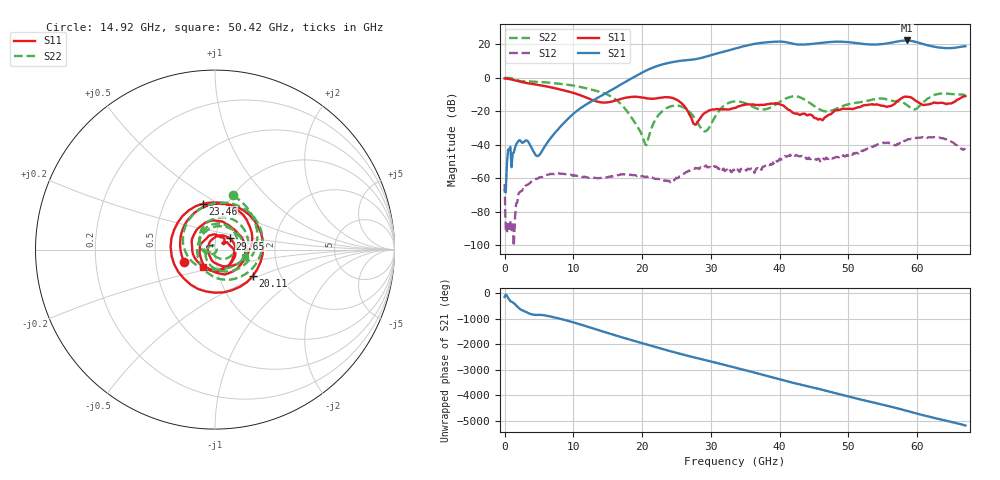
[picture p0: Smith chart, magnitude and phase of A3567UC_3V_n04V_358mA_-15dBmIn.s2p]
! MARKI MICROWAVE INC.
! Date:  4/20/2021
! Model Number:  A-3567UC
! Description:  2-port Small Signal S-parameter data for A-3567UC
! Frequency Range:  10 MHz to 67 GHz
! Port Configuration:  PORT 1: Input
!  PORT 2: Output
! Bias Condition: Vd = +3V, Vg = -0.4V, Id = 358mA
! A-3567UC s2p files are only valid for small signal conditions (below -10 dBm input power)
# Hz S  dB  R 50
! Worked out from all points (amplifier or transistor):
!   401 points, 10 MHz to 67 GHz, reference 50 ohm
!   highest |S21| = 22.3 dB at 58.46 GHz (marker M1)
!   |S21| within 3 dB of that: 35.21 GHz to 61.62 GHz (26.41 GHz wide, 54.5 % of centre)
!   unconditionally stable (mu >= 1): 178.7 MHz to end of sweep
!   at 11.06 GHz: K = 2250.85, MAG = -16.2 dB, |S12| = -58.7 dB
!   at 33.51 GHz: K = 40.23, MAG = 17.7 dB, |S12| = -56.0 dB
!   at 67 GHz: K = 6.21, MAG = 19.6 dB, |S12| = -42.2 dB
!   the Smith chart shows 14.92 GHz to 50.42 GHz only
!   S11 on the Smith chart (normalised r, x): 14.92 GHz: 0.70, -0.10; 20.11 GHz: 1.44, -0.46; 23.46 GHz: 0.77, +0.42; 29.65 GHz: 1.17, +0.15; 50.42 GHz: 0.86, -0.17
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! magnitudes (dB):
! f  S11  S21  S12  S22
! 10 MHz  -0.4  -67.1  -63.4  0.0
! 512.4 MHz  -0.6  -42.9  -85.6  0.0
! 2.02 GHz  -2.0  -37.7  -69.4  -1.6
! 4.867 GHz  -4.2  -46.7  -60.0  -2.4
! 11.23 GHz  -10.7  -17.6  -59.0  -5.6
! 14.92 GHz  -14.7  -8.8  -59.4  -9.9
! 20.11 GHz  -11.8  3.3  -58.7  -35.7
! 20.78 GHz  -12.3  4.7  -59.2  -38.0
! 22.45 GHz  -12.0  7.4  -60.5  -21.9
! 23.46 GHz  -11.5  8.5  -61.5  -18.3
! 25.8 GHz  -15.4  10.3  -57.9  -17.2
! 27.64 GHz  -27.8  11.1  -54.3  -24.1
! 29.65 GHz  -19.6  13.1  -53.3  -30.4
! 33.51 GHz  -17.9  17.4  -56.0  -14.1
! 39.7 GHz  -15.5  21.6  -50.0  -15.2
! 42.21 GHz  -21.3  20.1  -46.5  -11.0
! 44.73 GHz  -22.4  20.3  -47.8  -16.0
! 50.42 GHz  -18.6  21.1  -45.5  -15.3
! 55.95 GHz  -17.0  20.8  -39.1  -13.4
! 58.46 GHz  -11.3  22.3  -37.2  -16.2
! 61.14 GHz  -16.1  19.8  -35.8  -13.7
! 67 GHz  -10.9  18.9  -42.2  -10.2
